FUNCTION_BLOCK Example30_incoming //2x1 flyways 1 xbot (actual physical) with border 1 on the bottom edge of the 2 flyways - GetBorderStatus, ReadNumIncomingXbots, GetIncomingXbots
VAR_INPUT
	Execute : BOOL;
END_VAR
VAR_OUTPUT
	Done : BOOL;
END_VAR
VAR_IN_OUT
	PM_Controller : PMControllerType;	// the planar motor controller to use
END_VAR
VAR
	PMC_GetBorderStatus1 : PMC_GetBorderStatus;
	PMC_ReadNumIncomingXbots1: PMC_ReadNumIncomingXbots;
	num_incoming : USINT;
	processing_new_xbot : BOOL;
	PMC_GetIncomingXbots1 : PMC_GetIncomingXbots;
	nXbots : USINT;
	XbotIDS : ARRAY[0..149] OF USINT;
	BorderIDs : ARRAY[0..149] OF USINT;
	PMC_XYMotion1 : PMC_XYMotion;
	PMC_XYMotion2 : PMC_XYMotion;
	PMC_XYMotion3 : PMC_XYMotion;
END_VAR

//2x1 flyways 1 xbot (actual physical) with border 1 on the bottom edge of the 2 flyways - GetBorderStatus, ReadNumIncomingXbots, GetIncomingXbots
//additional user controlled PMC with 2x1 flyways with border 1 on the top edge, xbot starts on the user controlled PMC

//reset new xbot flag
IF(NOT(Execute))THEN
	processing_new_xbot := FALSE;
END_IF;

//verify status of the boundary 
PMC_GetBorderStatus1(Execute := Execute,BorderID := 1,PM_Controller := PM_Controller);

//wait until an xbot shows up on the boundary (user needs to manually move xbot over boundary using the other PMC)
PMC_ReadNumIncomingXbots1(Enable := PMC_GetBorderStatus1.Done AND PMC_GetBorderStatus1.State = 2,nXbots => num_incoming,PM_Controller := PM_Controller);
IF(num_incoming > 0 AND NOT(processing_new_xbot))THEN
	processing_new_xbot := TRUE;
END_IF;

//get ID of the incoming xbot
PMC_GetIncomingXbots1(Execute := processing_new_xbot,nXbots => nXbots,XbotIDs => XbotIDS,BorderIDs => BorderIDs,PM_Controller := PM_Controller);

//move xbot around the PLC controlled flyways
PMC_XYMotion1(Execute := PMC_GetIncomingXbots1.Done,XbotID := XbotIDS[0],PosX := 0.06,PosY := 0.18,PM_Controller := PM_Controller);
PMC_XYMotion2(Execute := PMC_XYMotion1.Done,XbotID := XbotIDS[0],PosX := 0.42,PosY := 0.18,PM_Controller := PM_Controller);

//move xbot back over the boundary
PMC_XYMotion3(Execute := PMC_XYMotion2.Done,XbotID := XbotIDS[0],PosX := 0.36,PosY := -0.12,PM_Controller := PM_Controller);

Done := PMC_XYMotion3.Done;
IF(Done)THEN
	processing_new_xbot := FALSE;
END_IF;

END_FUNCTION_BLOCK
